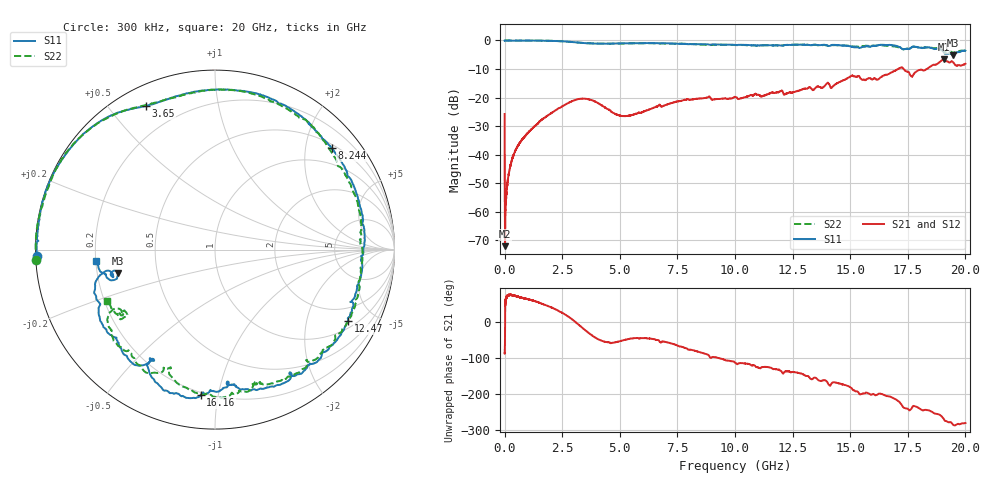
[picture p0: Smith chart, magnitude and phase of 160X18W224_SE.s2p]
!{160X18W224_SE}
!Johanson Technology Inc.
!www.johansontechnology.com
!Test Board Conditions:
!Substrate Type  RO4350B
!Substrate Thickness  21 mil
!Substrate Dk  3.66
!TL Type: GCPW
!TL Trace Width  40 mil
!TL Gap  20 mil
!PART MODE SINGLE ENDED (AKA BYPASS)
!DUT TOPOLOGY	SERIES-SHUNT
!Mounting Pad LxW  120x40 mil
! Created Wed Oct 27 11:08:00 2021
# hz S ma R 50
! 2 Port Network Data from SP1.SP block
! freq  magS11  angS11  magS21  angS21  magS12  angS12  magS22  angS22
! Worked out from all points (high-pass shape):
!   20001 points, 300 kHz to 20 GHz, reference 50 ohm
!   highest |S21| = -6.55 dB at 19.07 GHz (marker M1); lowest = -72.0 dB at 20.3 MHz (marker M2)
!   |S21| within 3 dB of the highest: 17.18 GHz to 17.27 GHz (93.98 MHz wide, 0.546 % of centre); 18.4 GHz to end of sweep
!   lowest |S11| = -5.1 dB at 19.45 GHz (marker M3), VSWR 3.49, Z = 14.5 - j5.49 ohm
!   |S11| at or under -10 dB: nowhere
!   |S22| runs from -4.4 to 0.0 dB; largest |S21 - S12| = 0.012
!   S11 on the Smith chart (normalised r, x): 300 kHz: 0.00, -0.02; 3.65 GHz: 0.08, +0.63; 8.244 GHz: 0.58, +2.55; 12.47 GHz: 1.29, -3.53; 16.16 GHz: 0.18, -0.89; 20 GHz: 0.20, -0.04
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300000  0.9938 -178.1  0.05164 -86.3  0.05174 -87.2  0.9986 -176.6
2.03e7  0.9952 179.7  0.0002505 -14.7  0.0002738 -10.3  1 179.7
1.043e8  0.9928 178.2  0.002586 72.4  0.002764 71.4  0.9999 178.1
1.883e8  0.9927 176.7  0.004815 75.8  0.004853 76.8  0.9986 176.8
3.293e8  0.994 174.1  0.008459 76.6  0.008435 76.4  0.9991 174.2
7.893e8  0.9966 166.0  0.01895 68.2  0.01905 68.2  0.9938 166.2
1.8783e9  0.9851 146.0  0.04873 46.0  0.04879 46.0  0.9885 146.8
3.3343e9  0.9061 119.8  0.09568 -12.9  0.09591 -12.9  0.9091 119.8
3.6503e9  0.8877 115.6  0.0932 -29.7  0.09341 -29.6  0.8919 115.2
5.1273e9  0.8882 93.9  0.04741 -50.4  0.04785 -50.3  0.8836 97.1
6.6673e9  0.8953 67.7  0.07182 -49.5  0.07183 -49.8  0.8894 70.5
8.2443e9  0.8617 41.1  0.09419 -79.1  0.09343 -79.0  0.8583 45.5
1.00003e10  0.8348 10.5  0.1028 -112.3  0.1035 -112.2  0.8295 16.4
1.24693e10  0.8416 -28.3  0.1215 -138.8  0.1196 -138.5  0.8398 -20.2
1.33343e10  0.8291 -44.1  0.141 -159.3  0.1414 -158.7  0.8259 -35.9
1.50583e10  0.778 -80.8  0.2409 175.9  0.2426 175.1  0.7896 -70.9
1.61603e10  0.8141 -95.7  0.2071 157.4  0.2065 157.6  0.8146 -84.0
1.66673e10  0.8343 -106.2  0.2587 153.1  0.2559 155.1  0.8082 -95.8
1.84253e10  0.753 -147.6  0.3384 113.4  0.3409 113.3  0.7594 -138.0
1.90653e10  0.6126 -169.0  0.4703 89.1  0.4683 89.2  0.6371 -149.0
1.94523e10  0.5549 -166.3  0.4221 74.2  0.418 74.0  0.6078 -145.6
2e10  0.6637 -175.0  0.3908 78.4  0.3908 77.4  0.6653 -155.0
